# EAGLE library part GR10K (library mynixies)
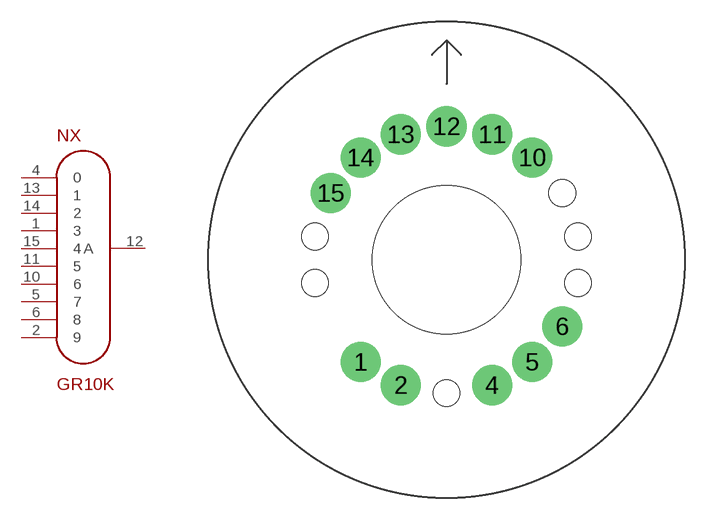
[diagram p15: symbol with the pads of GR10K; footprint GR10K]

Designator prefix NX

## GR10K  [GR10K]
1  3  pas
2  9  pas
4  0  pas
5  7  pas
6  8  pas
10  6  pas
11  5  pas
12  A  pas
13  1  pas
14  2  pas
15  4  pas

## Footprint GR10K (pad centres in mm)
drill 1.829: 1 -5.861,-6.985; 2 -3.119,-8.569; 4 3.119,-8.569; 5 5.861,-6.985; 6 7.897,-4.559; 10 5.861,6.985; 11 3.119,8.569; 12 0,9.119; 13 -3.119,8.569; 14 -5.861,6.985; 15 -7.897,4.559
hole 1.829 at 0,-9.119
hole 1.829 at 8.98,-1.583
hole 1.829 at 8.98,1.583
hole 1.829 at 7.897,4.559
hole 1.829 at -8.98,1.583
hole 1.829 at -8.98,-1.583
hole 10.16 at 0,0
